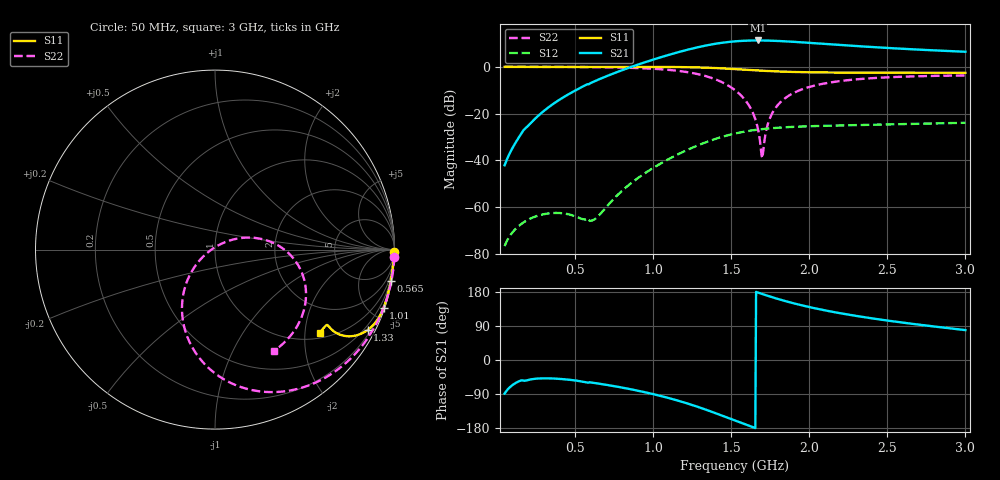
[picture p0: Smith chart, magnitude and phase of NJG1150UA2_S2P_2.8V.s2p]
!	Created	Tue	Apr	17	16:09:35	2012
#	hz	S	ma	R	50
!	2	Port	Network	Data	from	SP1.SP	block
!	freq	magS11	angS11	magS21	angS21	magS12	angS12	magS22	angS22
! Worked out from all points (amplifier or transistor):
!   591 points, 50 MHz to 3 GHz, reference 50 ohm
!   highest |S21| = 11.2 dB at 1.67 GHz (marker M1)
!   |S21| within 3 dB of that: 1.281 GHz to 2.449 GHz (1.169 GHz wide, 62.7 % of centre)
!   unconditionally stable (mu >= 1): 566.3 MHz to 976.3 MHz; 1.49 GHz to end of sweep
!   at 540 MHz: K = 0.72, MSG = 28.0 dB, |S12| = -64.8 dB
!   at 1.525 GHz: K = 1.01, MAG = 19.2 dB, |S12| = -28.5 dB
!   at 3 GHz: K = 1.28, MAG = 12.0 dB, |S12| = -23.9 dB
!   lowest NFmin = 0.21 dB at 530 MHz
!   S11 on the Smith chart (normalised r, x): 50 MHz: open; 565 MHz: 0, -11; 1.01 GHz: 0.11, -5.97; 1.33 GHz: 0.34, -4.01; 3 GHz: 1.15, -2.38
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5e7  0.9965 -0.9  0.00791 -88.6  0.0001482 88.4  0.9999 -2.3
1.3e8  0.9962 -2.3  0.02717 -58.5  0.000373 87.5  0.9994 -6.1
2.55e8  0.9955 -4.5  0.08377 -49.2  0.00065 86.9  0.9977 -12.0
5.45e8  0.9946 -9.6  0.3724 -56.6  0.0005664 116.2  0.987 -26.9
5.65e8  0.9945 -10.0  0.4018 -57.9  0.0005474 125.9  0.9855 -28.0
6.35e8  0.9944 -11.3  0.5064 -61.2  0.000586 165.8  0.9811 -32.0
8.25e8  0.9948 -14.9  0.9017 -74.6  0.002635 -151.5  0.9566 -44.2
1.01e9  0.9939 -19.0  1.454 -90.9  0.007226 -154.8  0.9045 -58.8
1.035e9  0.9934 -19.6  1.544 -93.4  0.008097 -156.1  0.8937 -61.1
1.18e9  0.9854 -23.4  2.13 -109.7  0.01459 -166.5  0.8042 -76.0
1.33e9  0.9608 -27.8  2.806 -129.8  0.02393 178.3  0.6428 -94.9
1.425e9  0.9324 -30.5  3.195 -144.2  0.0307 166.7  0.4975 -108.7
1.525e9  0.8933 -32.7  3.493 -159.8  0.0376 153.8  0.3173 -124.3
1.62e9  0.8537 -34.0  3.631 -174.4  0.04316 141.6  0.1394 -140.8
1.67e9  0.8345 -34.4  3.649 178.2  0.04555 135.5  0.05057 -155.8
1.7e9  0.8239 -34.5  3.643 174.0  0.04679 132.0  0.01117 113.7
1.74e9  0.811 -34.5  3.621 168.6  0.04826 127.6  0.06705 37.1
1.79e9  0.7973 -34.5  3.572 162.3  0.04979 122.4  0.1404 26.1
2.02e9  0.7616 -33.9  3.213 137.9  0.05408 103.1  0.3861 0.0
2.225e9  0.7515 -34.0  2.881 121.5  0.05624 90.8  0.5084 -16.1
2.51e9  0.7473 -35.1  2.514 103.6  0.05886 78.2  0.5979 -33.9
3e9  0.7441 -38.4  2.093 78.9  0.06382 61.8  0.6528 -59.9
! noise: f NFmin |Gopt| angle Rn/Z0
5e+07  0.4725  0.9545  2.794  3.387
3.75e+08  0.2305  0.8961  6.159  0.741
7.05e+08  0.2267  0.8626  10.07  0.5147
1.03e+09  0.2723  0.8356  14  0.4627
1.36e+09  0.3337  0.8084  18.06  0.4391
1.685e+09  0.4017  0.7814  22.07  0.4238
2.015e+09  0.4749  0.754  26.13  0.4111
2.34e+09  0.5504  0.7272  30.1  0.3999
2.67e+09  0.6302  0.7007  34.08  0.3896
3e+09  0.7141  0.6752  37.98  0.3811
